[IBIS Ver]   3.2
[File Name]   sprm429.ibs
[File Rev]   1.0
[Date]   November 3, 2003
[Source]   File originated at Texas Instruments
[Copyright]   (c) 2003, Texas Instruments Inc.
[Component]   f28235pgf
[Manufacturer] Texas Instruments
[Package]
| Variable   Typ   Min   Max
R_pkg   0.198   0.1909   0.2047
L_pkg   8.904e-09   8.346e-09   9.905e-09
C_pkg   1.561e-12   1.156e-12   1.834e-12
[Pin] signal_name   model_name   R_pin   L_pin   C_pin
1   GPIO[30]   BC3325CFHYPU   0.1921  9.905e-09  1.489e-12
2   GPIO[29]   BC3325CFHYPU   0.1951  9.662e-09  1.834e-12
3   VSS   NC   0.198   9.558e-09  1.805e-12
4   VDD   NC   0.2006  9.473e-09  1.771e-12
5   GPIO[0]   BC3350AFHYPU   0.2031  9.41e-09   1.706e-12
6   GPIO[1]   BC3350AFHYPU   0.2036  9.308e-09  1.669e-12
7   GPIO[2]   BC3350AFHYPU   0.2017  9.182e-09  1.673e-12
8   VSS   NC   0.2002  9.071e-09  1.647e-12
9   VDDIO   NC   0.1989  8.977e-09  1.625e-12
10   GPIO[3]   BC3350AFHYPU   0.1977  8.88e-09   1.606e-12
11   GPIO[4]   BC3350AFHYPU   0.1967  8.794e-09  1.581e-12
12   GPIO[5]   BC3350AFHYPU   0.1961  8.721e-09  1.56e-12
13   GPIO[6]   BC3350AFHYPU   0.1955  8.646e-09  1.544e-12
14   VSS   NC   0.195   8.579e-09  1.521e-12
15   VDD   NC   0.1949  8.524e-09  1.503e-12
16   GPIO[7]   BC3350AFHYPU   0.1948  8.469e-09  1.489e-12
17   GPIO[8]   BC3350AFHYPU   0.1948  8.424e-09  1.468e-12
18   GPIO[9]   BC3350AFHYPU   0.1952  8.388e-09  1.452e-12
19   GPIO[10]   BC3350AFHYPU   0.1954  8.359e-09  1.442e-12
20   GPIO[11]   BC3350AFHYPU   0.196   8.346e-09  1.424e-12
21   GPIO[12]   BC3350AFHYPU   0.1967  8.36e-09   1.411e-12
22   VSS   NC   0.1975  8.421e-09  1.16e-12
23   VDD   NC   0.198   8.429e-09  1.156e-12
24   GPIO[13]   BC3350AFHYPU   0.1973  8.376e-09  1.412e-12
25   GPIO[14]   BC3350AFHYPU   0.1971  8.373e-09  1.43e-12
26   GPIO[15]   BC3350AFHYPU   0.197   8.398e-09  1.442e-12
27   GPIO[16]   BC3350AFHYPU   0.197   8.435e-09  1.457e-12
28   GPIO[17]   BC3350AFHYPU   0.1974  8.484e-09  1.476e-12
29   VDD   NC   0.1977  8.542e-09  1.493e-12
30   VSS   NC   0.1984  8.61e-09   1.5e-12
31   VDD1A18   NC   0.1982  8.656e-09  1.517e-12
32   VSS1AGND   NC   0.1989  8.731e-09  1.548e-12
33   VSSA2   NC   0.2001  8.817e-09  1.558e-12
34   VDDA2   NC   0.1999  8.873e-09  1.577e-12
35   ADCINA[7]   NC   0.2013  8.967e-09  1.609e-12
36   ADCINA[6]   NC   0.2027  9.071e-09  1.622e-12
37   ADCINA[5]   NC   0.2027  9.139e-09  1.641e-12
38   ADCINA[4]   NC   0.2047  9.255e-09  1.665e-12
39   ADCINA[3]   NC   0.2047  9.341e-09  1.652e-12
40   ADCINA[2]   NC   0.2031  9.409e-09  1.689e-12
41   ADCINA[1]   NC   0.1983  9.422e-09  1.757e-12
42   ADCINA[0]   NC   0.1956  9.501e-09  1.801e-12
43   ADCLO   NC   0.1933  9.619e-09  1.832e-12
44   VSSAIO   NC   0.1909  9.876e-09  1.489e-12
45   VDDAIO   NC   0.1921  9.905e-09  1.489e-12
46   ADCINB[0]   NC   0.1951  9.662e-09  1.834e-12
47   ADCINB[1]   NC   0.198   9.558e-09  1.805e-12
48   ADCINB[2]   NC   0.2006  9.473e-09  1.771e-12
49   ADCINB[3]   NC   0.2031  9.41e-09   1.706e-12
50   ADCINB[4]   NC   0.2036  9.308e-09  1.669e-12
51   ADCINB[5]   NC   0.2017  9.182e-09  1.673e-12
52   ADCINB[6]   NC   0.2002  9.071e-09  1.647e-12
53   ADCINB[7]   NC   0.1989  8.977e-09  1.625e-12
54   ADCREFIN   NC   0.1977  8.88e-09   1.606e-12
55   ADCREFM   NC   0.1967  8.794e-09  1.581e-12
56   ADCREFP   NC   0.1961  8.721e-09  1.56e-12
57   ADCRESEXT   NC   0.1955  8.646e-09  1.544e-12
58   VSS2AGND   NC   0.195   8.579e-09  1.521e-12
59   VDD2A18   NC   0.1949  8.524e-09  1.503e-12
60   VSS   NC   0.1948  8.469e-09  1.489e-12
61   VDD   NC   0.1948  8.424e-09  1.468e-12
62   GPIO[18]   BC3350AFHYPU   0.1952  8.388e-09  1.452e-12
63   GPIO[19]   BC3350AFHYPU   0.1954  8.359e-09  1.442e-12
64   GPIO[20]   BC3350AFHYPU   0.196   8.346e-09  1.424e-12
65   GPIO[21]   BC3350AFHYPU   0.1967  8.36e-09   1.411e-12
66   GPIO[22]   BC3350AFHYPU   0.1975  8.421e-09  1.16e-12
67   GPIO[23]   BC3350AFHYPU   0.198   8.429e-09  1.156e-12
68   GPIO[24]   BC3350AFHYPU   0.1973  8.376e-09  1.412e-12
69   GPIO[25]   BC3350AFHYPU   0.1971  8.373e-09  1.43e-12
70   VSS   NC   0.197   8.398e-09  1.442e-12
71   VDDIO   NC   0.197   8.435e-09  1.457e-12
72   GPIO[26]   BC3350AFHYPU   0.1974  8.484e-09  1.476e-12
73   GPIO[27]   BC3350AFHYPU   0.1977  8.542e-09  1.493e-12
74   GPIO[32]   BC3350AFHYPU   0.1984  8.61e-09   1.5e-12
75   GPIO[33]   BC3350AFHYPU   0.1982  8.656e-09  1.517e-12
76   TDI   IC33FFSHYPU   0.1989  8.731e-09  1.548e-12
77   TDO   OC3325CF   0.2001  8.817e-09  1.558e-12
78   TRSTN   IC33FFSHYPD   0.1999  8.873e-09  1.577e-12
79   TMS   IC33FFSHYPU   0.2013  8.967e-09  1.609e-12
80   XRSN   BC3350BFODHYPU  0.2027  9.071e-09  1.622e-12
81   TEST1   NC   0.2027  9.139e-09  1.641e-12
82   TEST2   NC   0.2047  9.255e-09  1.665e-12
83   VSS   NC   0.2047  9.341e-09  1.652e-12
84   VDD3VFL   NC   0.2031  9.409e-09  1.689e-12
85   EMU0   BC3325CFHYPU   0.1983  9.422e-09  1.757e-12
86   EMU1   BC3325CFHYPU   0.1956  9.501e-09  1.801e-12
87   TCK   IC33FFSHYPU   0.1933  9.619e-09  1.832e-12
88   GPIO[48]   BC3325CFHYPU   0.1909  9.876e-09  1.489e-12
89   GPIO[49]   BC3325CFHYPU   0.1921  9.905e-09  1.489e-12
90   GPIO[50]   BC3325CFHYPU   0.1951  9.662e-09  1.834e-12
91   GPIO[51]   BC3325CFHYPU   0.198   9.558e-09  1.805e-12
92   VSS   NC   0.2006  9.473e-09  1.771e-12
93   VDDIO   NC   0.2031  9.41e-09   1.706e-12
94   GPIO[52]   BC3325CFHYPU   0.2036  9.308e-09  1.669e-12
95   GPIO[53]   BC3325CFHYPU   0.2017  9.182e-09  1.673e-12
96   GPIO[54]   BC3325CFHYPU   0.2002  9.071e-09  1.647e-12
97   GPIO[55]   BC3325CFHYPU   0.1989  8.977e-09  1.625e-12
98   GPIO[56]   BC3325CFHYPU   0.1977  8.88e-09   1.606e-12
99   GPIO[57]   BC3325CFHYPU   0.1967  8.794e-09  1.581e-12
100  GPIO[58]   BC3325CFHYPU   0.1961  8.721e-09  1.56e-12
101  VDD   NC   0.1955  8.646e-09  1.544e-12
102  X2   NC   0.195   8.579e-09  1.521e-12
103  VSS   NC   0.1949  8.524e-09  1.503e-12
104  X1   NC   0.1948  8.469e-09  1.489e-12
105  XCLKIN   IC33FFSHY   0.1948  8.424e-09  1.468e-12
106  VSS   NC   0.1952  8.388e-09  1.452e-12
107  VDDIO   NC   0.1954  8.359e-09  1.442e-12
108  VSS   NC   0.196   8.346e-09  1.424e-12
109  VDD   NC   0.1967  8.36e-09   1.411e-12
110  GPIO[59]   BC3325CFHYPU   0.1975  8.421e-09  1.16e-12
111  GPIO[60]   BC3325CFHYPU   0.198   8.429e-09  1.156e-12
112  GPIO[61]   BC3325CFHYPU   0.1973  8.376e-09  1.412e-12
113  GPIO[62]   BC3325CFHYPU   0.1971  8.373e-09  1.43e-12
114  GPIO[63]   BC3325CFHYPU   0.197   8.398e-09  1.442e-12
115  GPIO[64]   BC3325CFHYPU   0.197   8.435e-09  1.457e-12
116  GPIO[65]   BC3325CFHYPU   0.1974  8.484e-09  1.476e-12
117  VDD   NC   0.1977  8.542e-09  1.493e-12
118  VSS   NC   0.1984  8.61e-09   1.5e-12
119  GPIO[66]   BC3325CFHYPU   0.1982  8.656e-09  1.517e-12
120  VSS   NC   0.1989  8.731e-09  1.548e-12
121  VDDIO   NC   0.2001  8.817e-09  1.558e-12
122  GPIO[67]   BC3325CFHYPU   0.1999  8.873e-09  1.577e-12
123  GPIO[68]   BC3325CFHYPU   0.2013  8.967e-09  1.609e-12
124  GPIO[69]   BC3325CFHYPU   0.2027  9.071e-09  1.622e-12
125  VSS   NC   0.2027  9.139e-09  1.641e-12
126  VDD   NC   0.2047  9.255e-09  1.665e-12
127  GPIO[70]   BC3325CFHYPU   0.2047  9.341e-09  1.652e-12
128  GPIO[71]   BC3325CFHYPU   0.2031  9.409e-09  1.689e-12
129  GPIO[72]   BC3325CFHYPU   0.1983  9.422e-09  1.757e-12
130  GPIO[73]   BC3325CFHYPU   0.1956  9.501e-09  1.801e-12
131  GPIO[74]   BC3325CFHYPU   0.1933  9.619e-09  1.832e-12
132  GPIO[75]   BC3325CFHYPU   0.1909  9.876e-09  1.489e-12
133  GPIO[76]   BC3325CFHYPU   0.1921  9.905e-09  1.489e-12
134  GPIO[77]   BC3325CFHYPU   0.1951  9.662e-09  1.834e-12
135  GPIO[78]   BC3325CFHYPU   0.198   9.558e-09  1.805e-12
136  GPIO[79]   BC3325CFHYPU   0.2006  9.473e-09  1.771e-12
137  GPIO[38]   BC3325CFHYPU   0.2031  9.41e-09   1.706e-12
138  XCLKOUT   BC3325CF   0.2036  9.308e-09  1.669e-12
139  VDD   NC   0.2017  9.182e-09  1.673e-12
140  VSS   NC   0.2002  9.071e-09  1.647e-12
141  GPIO[28]   BC3325CFHYPU   0.1989  8.977e-09  1.625e-12
142  GPIO[34]   BC3350AFHYPU   0.1977  8.88e-09   1.606e-12
143  VDDIO   NC   0.1967  8.794e-09  1.581e-12
144  VSS   NC   0.1961  8.721e-09  1.56e-12
145  GPIO[36]   BC3325CFHYPU   0.1955  8.646e-09  1.544e-12
146  VDD   NC   0.195   8.579e-09  1.521e-12
147  VSS   NC   0.1949  8.524e-09  1.503e-12
148  GPIO[35]   BC3325CFHYPU   0.1948  8.469e-09  1.489e-12
149  XRDN   BC3325CFHYPU   0.1948  8.424e-09  1.468e-12
150  GPIO[37]   BC3325CFHYPU   0.1952  8.388e-09  1.452e-12
151  GPIO[40]   BC3325CFHYPU   0.1954  8.359e-09  1.442e-12
152  GPIO[41]   BC3325CFHYPU   0.196   8.346e-09  1.424e-12
153  GPIO[42]   BC3325CFHYPU   0.1967  8.36e-09   1.411e-12
154  VDD   NC   0.1975  8.421e-09  1.16e-12
155  VSS   NC   0.198   8.429e-09  1.156e-12
156  GPIO[43]   BC3325CFHYPU   0.1973  8.376e-09  1.412e-12
157  GPIO[44]   BC3325CFHYPU   0.1971  8.373e-09  1.43e-12
158  GPIO[45]   BC3325CFHYPU   0.197   8.398e-09  1.442e-12
159  VDDIO   NC   0.197   8.435e-09  1.457e-12
160  VSS   NC   0.1974  8.484e-09  1.476e-12
161  GPIO[46]   BC3325CFHYPU   0.1977  8.542e-09  1.493e-12
162  GPIO[47]   BC3325CFHYPU   0.1984  8.61e-09   1.5e-12
163  GPIO[80]   BC3325CFHYPU   0.1982  8.656e-09  1.517e-12
164  GPIO[81]   BC3325CFHYPU   0.1989  8.731e-09  1.548e-12
165  GPIO[82]   BC3325CFHYPU   0.2001  8.817e-09  1.558e-12
166  VSS   NC   0.1999  8.873e-09  1.577e-12
167  VDD   NC   0.2013  8.967e-09  1.609e-12
168  GPIO[83]   BC3325CFHYPU   0.2027  9.071e-09  1.622e-12
169  GPIO[84]   BC3325CFHYPU   0.2027  9.139e-09  1.641e-12
170  VDDIO   NC   0.2047  9.255e-09  1.665e-12
171  VSS   NC   0.2047  9.341e-09  1.652e-12
172  GPIO[85]   BC3325CFHYPU   0.2031  9.409e-09  1.689e-12
173  GPIO[86]   BC3325CFHYPU   0.1983  9.422e-09  1.757e-12
174  GPIO[87]   BC3325CFHYPU   0.1956  9.501e-09  1.801e-12
175  GPIO[39]   BC3325CFHYPU   0.1933  9.619e-09  1.832e-12
176  GPIO[31]   BC3325CFHYPU   0.1909  9.876e-09  1.489e-12
| End of package information
|   Component BC3325CFHYPU
[Component]   BC3325CFHYPU
[Manufacturer]   Texas Instruments.
[Package]
| variable   typ   min   max
R_pkg   0.000   0.000   0.000
L_pkg   0.000H   0.000H   0.000H
C_pkg   0.000F   0.000F   0.000F
[Pin]  signal_name   model_name   R_pin   L_pin   C_pin
PAD   PAD   BC3325CFHYPU_3P3PU
| A   A   dummy
| GZ   GZ   dummy
| Y   Y   dummy
VSSS   VSSS   GND
VDDS   VDDS   POWER
[Model Selector]   BC3325CFHYPU
BC3325CFHYPU_2P5PU   cell  VDDS=2.75(TYP)  PI=0
BC3325CFHYPU_2P5PUZ   cell  VDDS=2.75(TYP)  PI=1
BC3325CFHYPU_3P3PU   cell  VDDS=3.3(TYP)  PI=0
BC3325CFHYPU_3P3PUZ   cell  VDDS=3.3(TYP)  PI=1
|   Component BC3350AFHYPU
[Component]   BC3350AFHYPU
[Manufacturer]   Texas Instruments.
[Package]
| variable   typ   min   max
R_pkg   0.000   0.000   0.000
L_pkg   0.000H   0.000H   0.000H
C_pkg   0.000F   0.000F   0.000F
[Pin]  signal_name   model_name   R_pin   L_pin   C_pin
PAD   PAD   BC3350AFHYPU_3P3PU
| A   A   dummy
| GZ   GZ   dummy
| Y   Y   dummy
VSSS   VSSS   GND
VDDS   VDDS   POWER
[Model Selector]  BC3350AFHYPU
BC3350AFHYPU_2P5PU   cell   VDDS=2.5V(typ)  PI=0
BC3350AFHYPU_2P5PUZ  cell   VDDS=2.5V(typ)  PI=1
BC3350AFHYPU_3P3PU   cell   VDDS=3.3V(typ)  PI=0
BC3350AFHYPU_3P3PUZ  cell   VDDS=3.3V(typ)  PI=1
|   Component OC3325CF
[Component]   OC3325CF
[Manufacturer]   Texas Instruments.
[Package]
| variable   typ   min   max
R_pkg   0.000   0.000   0.000
L_pkg   0.000H   0.000H   0.000H
C_pkg   0.000F   0.000F   0.000F
[Pin]  signal_name   model_name   R_pin   L_pin   C_pin
PAD   PAD   OC3325CF_3P3
| A   A   dummy
| GZ   GZ   dummy
VDDS   VDDS   POWER
VSSS   VSSS   GND
VSS   VSS   GND
[Model Selector]   OC3325CF
OC3325CF_2P5  cell VDDS=2.5V(typ)
OC3325CF_2P7  cell VDDS=2.75V(typ)
OC3325CF_3P3  cell VDDS=3.3V(typ)
|   Component IC33FFSHYPD
[Component]   IC33FFSHYPD
[Manufacturer]   Texas Instruments.
[Package]
| variable   typ   min   max
R_pkg   0.000   0.000   0.000
L_pkg   0.000H   0.000H   0.000H
C_pkg   0.000F   0.000F   0.000F
[Pin]  signal_name   model_name   R_pin   L_pin   C_pin
PAD   PAD   IC33FFSHYPD_3P3PD
| Y   Y   dummy
VSS   VSS   GND
VDDS   VDDS   POWER
[Model Selector]  IC33FFSHYPD
IC33FFSHYPD_2P7PD   cell with PI=0 and VDDS as 2.75(typ)
IC33FFSHYPD_2P7PDZ   cell with PI=1 and VDDS as 2.75(typ)
IC33FFSHYPD_3P3PD   cell with PI=0 and VDDS as 3.3(typ)
IC33FFSHYPD_3P3PDZ   cell with PI=1 and VDDS as 3.3(typ)
|   Component IC33FFSHYPU
[Component]   IC33FFSHYPU
[Manufacturer]   Texas Instruments.
[Package]
| variable   typ   min   max
R_pkg   0.000   0.000   0.000
L_pkg   0.000H   0.000H   0.000H
C_pkg   0.000F   0.000F   0.000F
[Pin]  signal_name   model_name   R_pin   L_pin   C_pin
PAD   PAD   IC33FFSHYPU_3P3PU
| Y   Y   dummy
VSS   VSS   GND
VDDS   VDDS   POWER
[Model Selector]  IC33FFSHYPU
IC33FFSHYPU_2P5PU   cell with PI=0 VDDS=2.5(typ)
IC33FFSHYPU_2P5PUZ   cell with PI=1 VDDS=2.5(typ)
IC33FFSHYPU_2P7PU   cell with PI=0 VDDS=2.7(typ)
IC33FFSHYPU_2P7PUZ   cell with PI=1 VDDS=2.7(typ)
IC33FFSHYPU_3P3PU   cell with PI=0 VDDS=3.3(typ)
IC33FFSHYPU_3P3PUZ   cell with PI=1 VDDS=3.3(typ)
|   Component BC3325CF
[Component]   BC3325CF
[Manufacturer]   Texas Instruments.
[Package]
| variable   typ   min   max
R_pkg   0.000   0.000   0.000
L_pkg   0.000H   0.000H   0.000H
C_pkg   0.000F   0.000F   0.000F
[Pin]  signal_name   model_name   R_pin   L_pin   C_pin
PAD   PAD   BC3325CF_3P3PU
| A   A   dummy
| GZ   GZ   dummy
| Y   Y   dummy
VSSS   VSSS   GND
VDDS   VDDS   POWER
[Model Selector]  BC3325CF
BC3325CF_2P5PU  cell   VDDS=2.75V(typ)
BC3325CF_3P3PU  cell   VDDS=3.30V(typ)
|   Component BC3350BFODHYPU
[Component]   BC3350BFODHYPU
[Manufacturer]   Texas Instruments.
[Package]
| variable   typ   min   max
R_pkg   0.000   0.000   0.000
L_pkg   0.000H   0.000H   0.000H
C_pkg   0.000F   0.000F   0.000F
[Pin]  signal_name   model_name   R_pin   L_pin   C_pin
PAD   PAD   BC3350BFODHYPU_3P3PU
| A   A   dummy
| GZ   GZ   dummy
| Y   Y   dummy
VSSS   VSSS   GND
VDDS   VDDS   POWER
[Model Selector]   BC3350BFODHYPU
BC3350BFODHYPU_2P5PU   cell   VDDS=2.75(TYP)
BC3350BFODHYPU_2P5PZ   cell   VDDS=2.75(TYP)
BC3350BFODHYPU_3P3PU   cell   VDDS=3.3(TYP)
BC3350BFODHYPU_3P3PZ   cell   VDDS=3.3(TYP)
|   Component IC33FFSHY
[Component]   IC33FFSHY
[Manufacturer]   Texas Instruments.
[Package]
| variable   typ   min   max
R_pkg   0.000   0.000   0.000
L_pkg   0.000H   0.000H   0.000H
C_pkg   0.000F   0.000F   0.000F
[Pin]  signal_name   model_name   R_pin   L_pin   C_pin
PAD   PAD   IC33FFSHY_3P3
| Y   Y   dummy
VSS   VSS   GND
VDDS   VDDS   POWER
[Model Selector]  IC33FFSHY
IC33FFSHY_2P5   cell with VDDS=2.5(NOM)
IC33FFSHY_2P7   cell with VDDS=2.7(NOM)
IC33FFSHY_3P3   cell with VDDS=3.3(NOM)
| Models and submodels in the file (30): BC3325CFHYPU_2P5PU (I/O), BC3325CFHYPU_2P5PUZ (I/O), BC3325CFHYPU_3P3PU (I/O), BC3325CFHYPU_3P3PUZ (I/O), BC3350AFHYPU_2P5PU (I/O), BC3350AFHYPU_2P5PUZ (I/O), BC3350AFHYPU_3P3PU (I/O), BC3350AFHYPU_3P3PUZ (I/O), OC3325CF_2P5 (3-state), OC3325CF_2P7 (3-state), OC3325CF_3P3 (3-state), IC33FFSHYPD_2P7PD (Input), IC33FFSHYPD_2P7PDZ (Input), IC33FFSHYPD_3P3PD (Input), IC33FFSHYPD_3P3PDZ (Input), IC33FFSHYPU_2P5PU (Input), IC33FFSHYPU_2P5PUZ (Input), IC33FFSHYPU_2P7PU (Input), IC33FFSHYPU_2P7PUZ (Input), IC33FFSHYPU_3P3PU (Input), IC33FFSHYPU_3P3PUZ (Input), BC3325CF_2P5PU (I/O), BC3325CF_3P3PU (I/O), BC3350BFODHYPU_2P5PU (I/O_open_drain), BC3350BFODHYPU_2P5PZ (I/O_open_drain), BC3350BFODHYPU_3P3PU (I/O_open_drain), BC3350BFODHYPU_3P3PZ (I/O_open_drain), IC33FFSHY_2P5 (Input), IC33FFSHY_2P7 (Input), IC33FFSHY_3P3 (Input)
